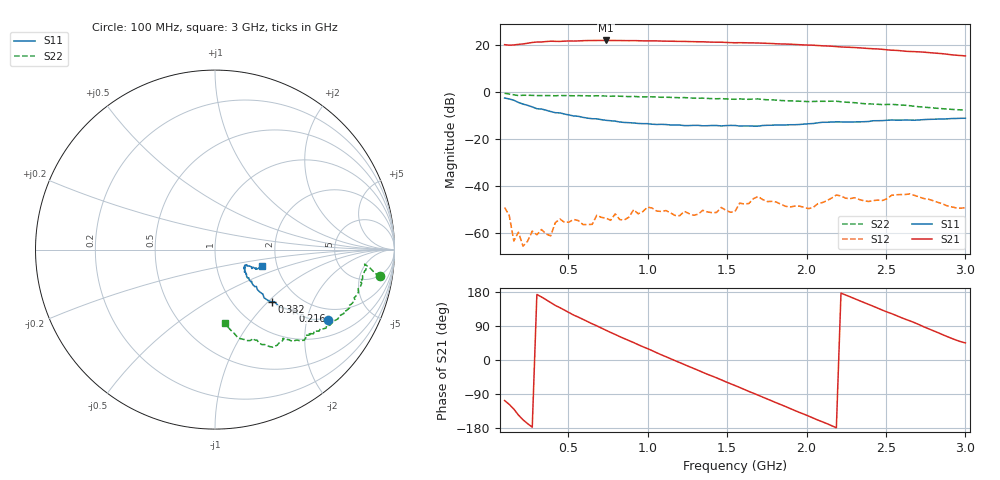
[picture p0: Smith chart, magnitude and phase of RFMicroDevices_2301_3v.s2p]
! RF Micro Devices
! RF2301
! Vcc = 3.0V
# HZ S MA R 50
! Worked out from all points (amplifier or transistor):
!   101 points, 100 MHz to 3 GHz, reference 50 ohm
!   highest |S21| = 21.8 dB at 738 MHz (marker M1)
!   |S21| within 3 dB of that: start of sweep to 2.302 GHz
!   unconditionally stable (mu >= 1): start of sweep to end of sweep
!   at 564 MHz: K = 6.38, MAG = 27.1 dB, |S12| = -54.6 dB
!   at 1.55 GHz: K = 7.60, MAG = 24.0 dB, |S12| = -50.7 dB
!   at 3 GHz: K = 18.76, MAG = 16.4 dB, |S12| = -49.1 dB
!   S11 on the Smith chart (normalised r, x): 100 MHz: 1.55, -2.70; 216 MHz: 1.60, -1.56; 332 MHz: 1.48, -1.07; 3 GHz: 1.67, -0.33
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1e8  0.7421 -31.9  10.03 -107.0  0.003528 -107.3  0.9323 -9.2
1.58e8  0.6654 -35.9  9.897 -129.5  0.0006909 -77.5  0.868 -6.7
2.16e8  0.5509 -38.0  10.41 -158.0  0.0005352 -7.9  0.8481 -7.0
2.74e8  0.4808 -41.7  11.17 -177.3  0.001116 38.6  0.8438 -8.0
3.32e8  0.4336 -42.7  11.43 166.4  0.001208 78.5  0.835 -10.0
4.19e8  0.3624 -42.8  11.81 144.0  0.001683 78.5  0.8269 -12.4
5.93e8  0.2884 -42.9  12.18 107.3  0.001538 25.1  0.8298 -17.5
7.38e8  0.2498 -40.8  12.32 78.5  0.002111 6.1  0.8167 -22.0
9.41e8  0.2144 -37.1  12.18 40.4  0.002599 6.0  0.7901 -27.5
1.086e9  0.2052 -35.2  11.96 13.8  0.002913 2.3  0.7686 -31.0
1.289e9  0.1951 -31.3  11.61 -22.1  0.002418 -19.8  0.7385 -36.8
1.463e9  0.19 -31.3  11.3 -52.2  0.003552 -32.2  0.7217 -40.6
1.55e9  0.194 -30.8  11.02 -67.3  0.002905 -14.1  0.6975 -41.5
1.666e9  0.1878 -28.6  10.93 -87.7  0.005439 -23.4  0.7037 -43.5
1.753e9  0.1957 -26.9  10.7 -102.9  0.004725 -51.1  0.6809 -47.7
1.898e9  0.2011 -26.9  10.25 -128.2  0.00363 -64.0  0.6438 -51.0
2.043e9  0.2137 -25.4  9.769 -153.4  0.00357 -49.8  0.6262 -52.4
2.159e9  0.2296 -25.5  9.312 -173.5  0.005621 -56.2  0.6352 -56.8
2.275e9  0.23 -26.3  8.816 166.7  0.00545 -74.4  0.5972 -62.4
2.536e9  0.2526 -25.5  7.654 122.3  0.006438 -83.5  0.5433 -68.9
2.739e9  0.2584 -24.5  6.96 87.5  0.005473 -120.1  0.4739 -77.4
3e9  0.2762 -19.1  5.79 45.1  0.003505 -112.6  0.4145 -82.4
